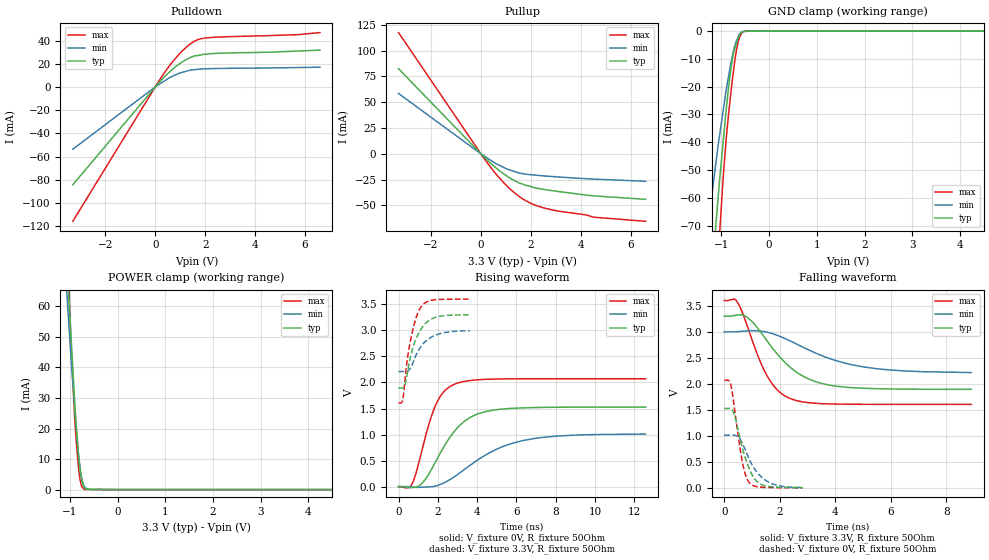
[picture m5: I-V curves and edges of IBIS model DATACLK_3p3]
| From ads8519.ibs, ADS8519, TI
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|   dataclk_3p3 Model
[Model]   DATACLK_3p3
Model_type   I/O
Polarity   Non-Inverting
Enable   Active-Low
Vinl = 0.6
Vinh = 1.65
Vmeas = 1.65
Vref = 1.65
Cref = 15pF
Rref = 50
|   typ   min   max
|   (nom PVT)   (Fast PVT)   (slow PVT)
| C_comp by Frequency method (F=29Mhz)
|Average
|C_comp   1.020e-11   9.004e-12   1.145e-11
|ON state : BUFFER OUTPUT TURNED HIGH
|C_comp   1.178e-11   1.045e-11   1.327e-11
|OFF state: BUFFER IN HIGH IMPEDANCE
|C_comp   8.614e-12   7.561e-12   9.627e-12
| C_comp by LC Tank method (L=1nH)
| Resonant frequency (Hz) 1.77e9   1.86e9   1.7e9
|Average
C_comp   9.050e-12   7.294e-12   9.775e-12
| Where nom  PVT is Nominal Process,  3.3V,  32C
|   Fast PVT is Strong Process,   3.6V,  -40C
|   Slow PVT is Weak Process,   3V,  92C
[Model Spec]
Vinl   0.6   0.6   0.6
Vinh   1.65   1.5   1.85
[Voltage Range]   3.3   3   3.6
|Ambient Temperature   25   85   -40
|Junction Temperature
[Temperature Range]   32   92   -40
[Pullup Reference]   3.3   3   3.6
[Pulldown Reference]   0   0   0
[Power Clamp Reference]   3.3   3   3.6
[GND Clamp Reference]   0   0   0
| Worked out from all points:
|   slope of the pulldown table from 0 to 0.495 V, typ, clamps not added: 43.8 ohm
|   slope of the pullup table from 0 to 0.495 V, typ, clamps not added: 43.7 ohm
|   GND clamp passes 1 mA (typ) near -0.60 V on its own axis
|   POWER clamp passes 1 mA (typ) near -0.71 V on its own axis
|   falling waveform, V_fixture 3.3V, R_fixture 50Ohm: 20-80 % time 1.47ns typ, 2.24ns min, 953ps max; typ from 3.3 V to 1.89 V
|   rising waveform, V_fixture 0V, R_fixture 50Ohm: 20-80 % time 1.62ns typ, 2.71ns min, 1.01ns max; typ from 0 V to 1.53 V
|   rising waveform, V_fixture 3.3V, R_fixture 50Ohm: 20-80 % time 685ps typ, 811ps min, 543ps max; typ from 1.89 V to 3.3 V
|   falling waveform, V_fixture 0V, R_fixture 50Ohm: 20-80 % time 496ps typ, 649ps min, 348ps max; typ from 1.53 V to 0.006 V
[Pulldown]
|   Voltage   I(typ)   I(min)   I(max)
-3.3V     -84.31mA   -53.64mA   -115.8mA
18mV      444.4uA    291.4uA    639.9uA
277.2mV   6.701mA    3.922mA    9.4mA
633.6mV   14.15mA    8.698mA    20.02mA
939.6mV   19.44mA    11.61mA    27.79mA
1.422V    25.54mA    14.6mA     37.33mA
1.706V    27.14mA    15.22mA    40.81mA
2.167V    28.64mA    15.76mA    42.53mA
5.774V    31.03mA    16.78mA    45.18mA
6.6V      31.76mA    17.04mA    46.89mA
[GND Clamp]
|   Voltage   I(typ)   I(min)   I(max)
-3.3V     -584.1mA   -414.2mA   -809.7mA
-1.354V   -119.8mA   -80.51mA   -170.2mA
-1.263V   -100.1mA   -67.22mA   -141.3mA
-1.204V   -87.43mA   -59.36mA   -123.4mA
-1.065V   -59.1mA    -40.67mA   -80.69mA
-1.036V   -53.25mA   -37.28mA   -72.46mA
-896.4mV  -27.83mA   -20.84mA   -38.17mA
-811.8mV  -15.1mA    -12.62mA   -23.96mA
-738mV    -7.485mA   -6.543mA   -13.16mA
-655.2mV  -2.997mA   -2.396mA   -4.432mA
-534mV    -211.9uA   -177.9uA   -273.7uA
6.6V      0A         0A         0A
[Pullup]
|   Voltage   I(typ)   I(min)   I(max)
-3.3V     82.52mA    58.52mA    117.5mA
172.8mV   -4.205mA   -2.782mA   -6.008mA
572.4mV   -12.96mA   -9.063mA   -18.68mA
939.6mV   -19.9mA    -13.52mA   -28.71mA
1.246V    -24.66mA   -16.34mA   -35.81mA
1.566V    -28.56mA   -18.78mA   -41.95mA
2.167V    -32.98mA   -20.64mA   -49.72mA
2.934V    -35.99mA   -22.15mA   -54.79mA
4.19V     -39.92mA   -24.09mA   -59.15mA
4.5V      -40.72mA   -24.48mA   -61.39mA
6.6V      -44.11mA   -26.61mA   -65.41mA
[POWER Clamp]
|   Voltage   I(typ)   I(min)   I(max)
-3.3V     870.4mA    741.8mA    1.056A
-1.069V   78.29mA    65.03mA    85.74mA
-1.013V   59.91mA    51.58mA    62.19mA
-972mV    48.41mA    41.73mA    44.95mA
-896.4mV  27.3mA     25.31mA    22mA
-871.2mV  21.33mA    20.66mA    16.38mA
-828mV    12.55mA    12.69mA    8.336mA
-792mV    6.899mA    7.562mA    3.495mA
-745.8mV  2.391mA    3.17mA     797.3uA
-702mV    692.9uA    1.082mA    83.89uA
-591mV    124.4uA    40.79uA    48.46uA
6.6V      0A         0A         0A
[Ramp]
R_load = 50
|   typ   min   max
dV/dt_r   0.916648/1.61486e-09   0.608017/2.7196e-09   1.24239/1.00505e-09
dV/dt_f   0.843862/1.47066e-09   0.473852/2.28556e-09   1.19615/9.52277e-10
[Falling Waveform]
V_fixture = 3.3V
V_fixture_min = 3V
V_fixture_max = 3.6V
R_fixture = 50Ohm
|   Time   V(typ)   V(min)   V(max)
0s        3.3V       3V         3.6V
425ps     3.318V     3.002V     3.606V
825ps     3.282V     3.018V     3.12V
1.2ns     3.073V     3.019V     2.556V
1.55ns    2.821V     2.993V     2.15V
1.95ns    2.548V     2.925V     1.864V
2.425ns   2.297V     2.812V     1.709V
3.375ns   2.028V     2.573V     1.624V
4.925ns   1.918V     2.334V     1.607V
8.9ns     1.894V     2.217V     1.606V
[Rising Waveform]
V_fixture = 0V
V_fixture_min = 0V
V_fixture_max = 0V
R_fixture = 50Ohm
|   Time   V(typ)   V(min)   V(max)
0s        2.612nV    3.03nV     2.328nV
675ps     -16.48mV   -7.179mV   43.48mV
875ps     -9.36mV    -13.63mV   240.1mV
1.2ns     64.52mV    -10.73mV   708.8mV
1.825ns   434.9mV    8.037mV    1.506V
2.25ns    728.4mV    61.11mV    1.798V
2.85ns    1.065V     192.4mV    1.966V
4.075ns   1.402V     524.1mV    2.052V
6.325ns   1.512V     884mV      2.07V
12.58ns   1.528V     1.01V      2.071V
[Rising Waveform]
V_fixture = 3.3V
V_fixture_min = 3V
V_fixture_max = 3.6V
R_fixture = 50Ohm
|   Time   V(typ)   V(min)   V(max)
0s        1.894V     2.21V      1.606V
200ps     1.894V     2.21V      1.643V
250ps     1.901V     2.21V      1.751V
350ps     1.981V     2.209V     2.129V
475ps     2.233V     2.221V     2.513V
600ps     2.478V     2.271V     2.787V
875ps     2.823V     2.51V      3.219V
1.125ns   3.011V     2.681V     3.436V
1.875ns   3.249V     2.907V     3.589V
3.625ns   3.297V     2.993V     3.599V
[Falling Waveform]
V_fixture = 0V
V_fixture_min = 0V
V_fixture_max = 0V
R_fixture = 50Ohm
|   Time   V(typ)   V(min)   V(max)
0s        1.527V     1.014V     2.068V
175ps     1.527V     1.013V     2.06V
250ps     1.52V      1.014V     1.955V
375ps     1.391V     1.013V     1.502V
625ps     826.1mV    887.7mV    579.4mV
750ps     597.2mV    742.9mV    278.6mV
875ps     406.5mV    584mV      123mV
1.175ns   125.2mV    304.5mV    25.08mV
1.575ns   28.88mV    119.4mV    8.597mV
2.825ns   6.075mV    8.363mV    1.921mV
